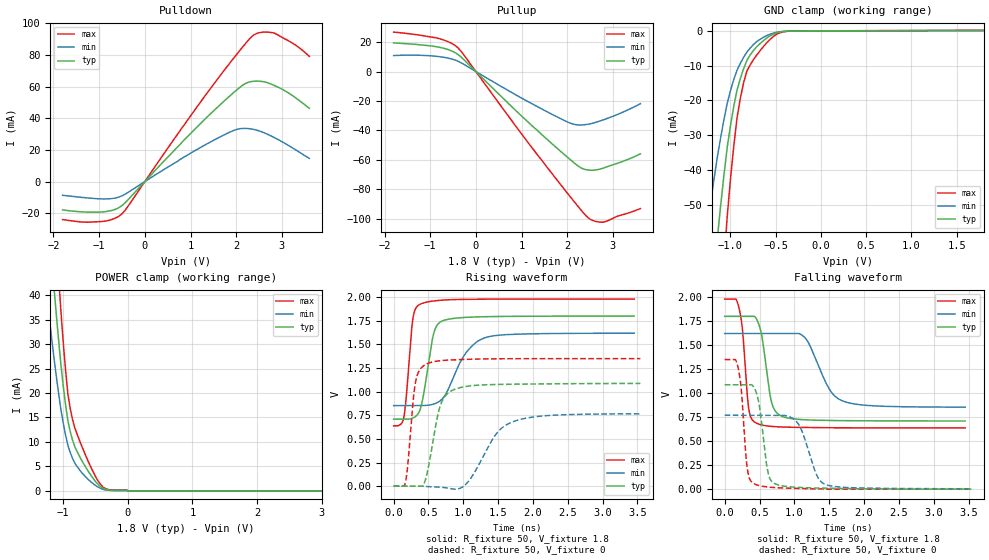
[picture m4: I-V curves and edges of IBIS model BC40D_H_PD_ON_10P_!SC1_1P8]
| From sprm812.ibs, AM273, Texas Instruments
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|   Model Cell BC40D_H_PD_ON_10P_!SC1_1P8
|BC40D_H_PD_ON_10P_!SC1_1P8
[Model]   BC40D_H_PD_ON_10P_!SC1_1P8
Model_type   I/O
Polarity   Non-Inverting
Enable   Active-Low
Vinl =  0.63
Vinh =  1.17
Cref =  15pF
Rref =  100.0000M
Vref =  0V
Vmeas =  0.9
C_comp   2.389419p   2.292106p   2.408415p
|[Input load] weak_pd_on
|[Output drive] fast
|[supplytol] 10
|[temp] ind
[Model Spec]
Vinl   0.63   0.567   0.693
Vinh   1.17   1.053   1.287
[Temperature Range]   25   125   -40
[Voltage Range]   1.8   1.62   1.98
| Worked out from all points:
|   slope of the pulldown table from 0 to 0.27 V, typ, clamps not added: 32.2 ohm
|   slope of the pullup table from 0 to 0.27 V, typ, clamps not added: 32.5 ohm
|   GND clamp passes 1 mA (typ) near -0.53 V on its own axis
|   POWER clamp passes 1 mA (typ) near -0.43 V on its own axis
|   rising waveform, R_fixture 50, V_fixture 1.8: 20-80 % time 145ps typ, 331ps min, 88.9ps max; typ from 0.708 V to 1.8 V
|   rising waveform, R_fixture 50, V_fixture 0: 20-80 % time 176ps typ, 382ps min, 101ps max; typ from 0 V to 1.09 V
|   falling waveform, R_fixture 50, V_fixture 1.8: 20-80 % time 130ps typ, 293ps min, 86ps max; typ from 1.8 V to 0.709 V
|   falling waveform, R_fixture 50, V_fixture 0: 20-80 % time 113ps typ, 213ps min, 82.8ps max; typ from 1.09 V to 0 V
| Nom Voltages:
|   VDD=1.1001, VDDS=1.8, VDDS18=1.8, ESD_BIASFET=0, VSS=0, VSSS=0
| Min Voltages:
|   VDD=0.99, VDDS=1.62, VDDS18=1.62, ESD_BIASFET=0, VSS=0, VSSS=0
| Max Voltages:
|   VDD=1.21, VDDS=1.98, VDDS18=1.98, ESD_BIASFET=0, VSS=0, VSSS=0
[POWER_clamp]
|   voltage   I(typ)   I(min)   I(max)
-1.8V     158.9mA    112.6mA    219.9mA
-1.255V   60.04mA    40.04mA    85.04mA
-1.145V   41.99mA    27.45mA    59.9mA
-1.109V   36.4mA     23.66mA    51.96mA
-1.073V   31.03mA    20.08mA    44.3mA
-1.036V   25.91mA    16.71mA    36.9mA
-927.3mV  14.27mA    9.297mA    19.77mA
-854.5mV  10.33mA    6.619mA    14.49mA
-454.5mV  1.273mA    741.7uA    1.94mA
-309.1mV  221.6uA    132.8uA    307.9uA
18.18mV   0A         0A         0A
3.6V      0A         0A         0A
[Pulldown]
|   voltage   I(typ)   I(min)   I(max)
-1.8V     -17.92mA   -8.674mA   -24.03mA
-927.3mV  -19.22mA   -10.99mA   -25.2mA
-654.5mV  -17.65mA   -10.46mA   -23.22mA
-490.9mV  -14.97mA   -8.904mA   -20.12mA
872.7mV   26.63mA    15.72mA    36.29mA
1.691V    49.7mA     28.87mA    68.58mA
2.127V    60.63mA    33.53mA    84.59mA
2.4V      63.43mA    32.85mA    92.9mA
2.618V    62.99mA    30.74mA    94.47mA
2.836V    60.69mA    27.76mA    93.76mA
3.273V    53.49mA    20.53mA    86.73mA
3.6V      46.26mA    14.64mA    79.12mA
[Pullup]
|   voltage   I(typ)   I(min)   I(max)
-1.8V     19.47mA    10.86mA    26.81mA
-818.2mV  16.61mA    10.18mA    22.5mA
-545.5mV  14.2mA     8.665mA    19.39mA
-381.8mV  11.35mA    6.855mA    15.77mA
1.036V    -31.31mA   -18.66mA   -43.94mA
1.909V    -55.72mA   -32.86mA   -78.99mA
2.182V    -62.87mA   -36.1mA    -89.59mA
2.345V    -66.12mA   -36.26mA   -95.76mA
2.455V    -66.95mA   -35.82mA   -99.33mA
2.618V    -66.9mA    -34.58mA   -101.8mA
2.782V    -65.72mA   -32.89mA   -102.4mA
3.6V      -55.92mA   -21.86mA   -93.15mA
[GND_clamp]
|   voltage   I(typ)   I(min)   I(max)
-1.8V     -270.2mA   -170.2mA   -430.1mA
-1.255V   -91.66mA   -55.91mA   -148.4mA
-1.145V   -59.91mA   -36.45mA   -97.1mA
-1.109V   -50.48mA   -30.83mA   -81.56mA
-1.073V   -41.73mA   -25.65mA   -67.06mA
-1.036V   -33.67mA   -20.93mA   -53.6mA
-927.3mV  -17.08mA   -11.35mA   -25.06mA
-854.5mV  -10.88mA   -7.623mA   -14.95mA
-781.8mV  -6.944mA   -4.955mA   -9.81mA
-636.4mV  -2.852mA   -1.883mA   -4.568mA
-381.8mV  -107.5uA   -91.83uA   -158.4uA
1.8V      101.9uA    59.86uA    152.6uA
[Ramp]
| variable   typ   min   max
dV/dt_f   0.664662/0.13254911n  0.4701722/0.29942463n 0.81361914/87.565727p
dV/dt_r 0.66395697/0.17823366n 0.48090772/0.39818705n 0.81798459/0.10141802n
R_load = 50
[Rising Waveform]
R_fixture = 50
V_fixture = 1.8
V_fixture_min = 1.62
V_fixture_max = 1.98
|   time   V(typ)   V(min)   V(max)
0s        708.4mV    851.3mV    637.7mV
145.4ps   708.4mV    851.3mV    724.8mV
179.5ps   708.4mV    851.3mV    929.6mV
273ps     720.2mV    851.3mV    1.753V
373.6ps   797.1mV    851.3mV    1.92V
571.3ps   1.604V     866.6mV    1.957V
694.4ps   1.745V     919.4mV    1.966V
1.017ns   1.783V     1.387V     1.974V
1.315ns   1.791V     1.569V     1.976V
3.453ns   1.798V     1.617V     1.977V
[Rising Waveform]
R_fixture = 50
V_fixture = 0
V_fixture_min = 0
V_fixture_max = 0
|   time   V(typ)   V(min)   V(max)
0s        0V         0V         0V
168.3ps   0V         0V         39.18mV
312ps     0V         0V         1.091V
465ps     90.38mV    -2.662mV   1.288V
661.8ps   832.5mV    -10.42mV   1.326V
859.8ps   1.019V     -30.72mV   1.335V
1.065ns   1.057V     42.98mV    1.341V
1.47ns    1.075V     550.3mV    1.346V
1.69ns    1.077V     674.8mV    1.347V
3.542ns   1.086V     764.7mV    1.348V
[Falling Waveform]
R_fixture = 50
V_fixture = 1.8
V_fixture_min = 1.62
V_fixture_max = 1.98
|   time   V(typ)   V(min)   V(max)
0s        1.798V     1.62V      1.978V
201.8ps   1.798V     1.62V      1.895V
257.1ps   1.798V     1.62V      1.645V
345.3ps   1.798V     1.62V      837mV
452.7ps   1.775V     1.62V      687.8mV
670.3ps   913.4mV    1.62V      653.2mV
808.4ps   762.5mV    1.62V      647.1mV
1.156ns   721.8mV    1.573V     642.3mV
1.696ns   713.1mV    917.3mV    638.4mV
3.453ns   709.3mV    853.6mV    637.1mV
[Falling Waveform]
R_fixture = 50
V_fixture = 0
V_fixture_min = 0
V_fixture_max = 0
|   time   V(typ)   V(min)   V(max)
0s        1.086V     769mV      1.348V
189.2ps   1.086V     769mV      1.275V
238.4ps   1.086V     769mV      1.036V
323.6ps   1.086V     769mV      220.9mV
428.8ps   1.049V     769mV      54.76mV
620.9ps   177.7mV    769mV      22.52mV
721.3ps   56.41mV    769mV      16.37mV
1.052ns   18.65mV    684.4mV    7.284mV
1.456ns   9.792mV    46.35mV    0V
3.542ns   0V         3.44mV     0V
